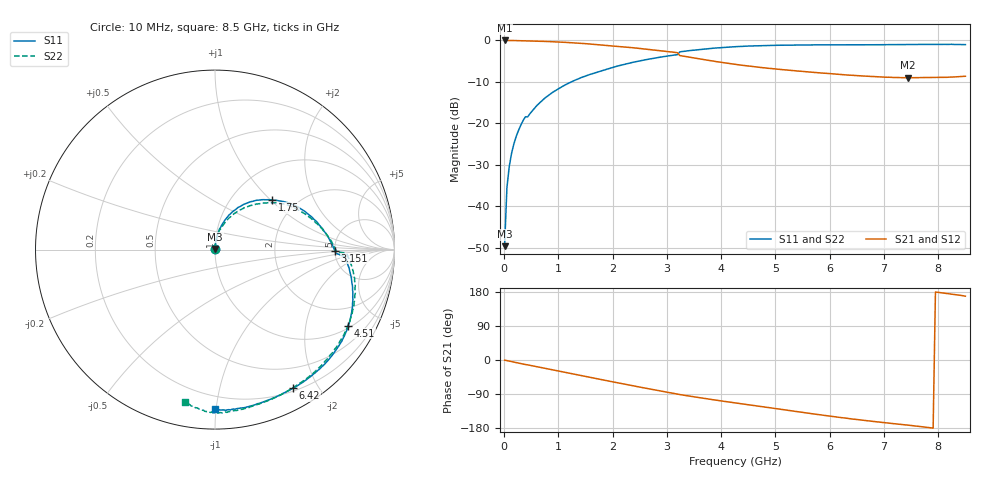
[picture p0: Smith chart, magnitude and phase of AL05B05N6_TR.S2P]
!AVX Corporation
!PN: AL05B05N6*TR
!Description: Air Core Inductor, 5.6nH, 6 Turns
!Agilent Technologies,E5071C,MY46102230,A.09.54
!Date: Mon Sep 03 16:21:16 2012
!Data & Calibration Information:
!Freq	S11:SOLT2(ON)	S21:SOLT2(ON)	S12:SOLT2(ON)	S22:SOLT2(ON)
# Hz S dB R 50
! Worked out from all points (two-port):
!   201 points, 10 MHz to 8.5 GHz, reference 50 ohm
!   highest |S21| = 0.00 dB at 10 MHz (marker M1); lowest = -9.0 dB at 7.439 GHz (marker M2)
!   |S21| within 3 dB of the highest: start of sweep to 3.197 GHz
!   lowest |S11| = -49.6 dB at 10 MHz (marker M3), VSWR 1.01, Z = 50.1 + j0.325 ohm
!   |S11| at or under -10 dB: start of sweep to 1.241 GHz
!   |S22| runs from -49.6 to -0.8 dB; largest |S21 - S12| = 0.0059
!   S11 on the Smith chart (normalised r, x): 10 MHz: 1.00, +0.01; 1.75 GHz: 1.52, +1.02; 3.151 GHz: 5.03, -0.11; 4.51 GHz: 1.09, -3.46; 6.42 GHz: 0.24, -1.69; 8.5 GHz: 0.12, -0.99
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1e7  -49.63 80.1  -0.00 -0.3  -0.04 -0.1  -49.62 79.5
5.245e7  -35.51 87.1  -0.01 -1.6  0.03 -1.7  -35.33 86.4
9.49e7  -30.47 85.7  -0.02 -2.9  -0.00 -2.9  -30.49 84.3
1.798e8  -25.01 83.0  -0.03 -5.5  -0.02 -5.5  -24.94 82.4
3.0715e8  -20.48 79.4  -0.06 -9.4  -0.05 -9.4  -20.45 79.0
3.9205e8  -18.43 77.5  -0.10 -11.9  -0.08 -12.0  -18.42 75.8
7.741e8  -13.68 68.1  -0.24 -22.6  -0.24 -22.7  -13.75 64.2
1.4533e9  -8.81 49.4  -0.73 -42.3  -0.72 -42.3  -8.86 45.3
1.75045e9  -7.52 41.0  -1.05 -50.9  -1.04 -50.9  -7.41 37.7
2.2174e9  -5.75 27.7  -1.58 -63.5  -1.57 -63.6  -5.62 24.1
2.85415e9  -4.09 8.2  -2.44 -81.2  -2.43 -81.2  -4.02 7.5
3.1513e9  -3.50 -0.5  -2.90 -89.1  -2.89 -89.2  -3.45 -0.0
3.2362e9  -2.78 -3.3  -3.63 -91.1  -3.63 -91.2  -2.70 -1.6
3.4909e9  -2.34 -9.7  -4.21 -97.1  -4.20 -97.1  -2.28 -7.3
4.255e9  -1.51 -25.3  -5.76 -113.1  -5.76 -113.2  -1.54 -23.5
4.5097e9  -1.35 -29.7  -6.18 -118.3  -6.19 -118.3  -1.40 -29.0
5.06155e9  -1.16 -38.8  -6.95 -129.3  -6.95 -129.3  -1.20 -41.5
5.6983e9  -1.06 -48.9  -7.70 -142.2  -7.69 -142.2  -1.09 -56.6
6.41995e9  -1.06 -60.5  -8.41 -155.8  -8.41 -155.8  -0.99 -72.6
7.09915e9  -1.02 -70.8  -8.88 -166.8  -8.88 -166.8  -0.85 -84.2
7.43875e9  -0.98 -75.6  -8.99 -171.9  -8.99 -171.8  -0.82 -88.6
8.5e9  -1.02 -89.9  -8.64 168.4  -8.64 168.4  -1.28 -101.0
